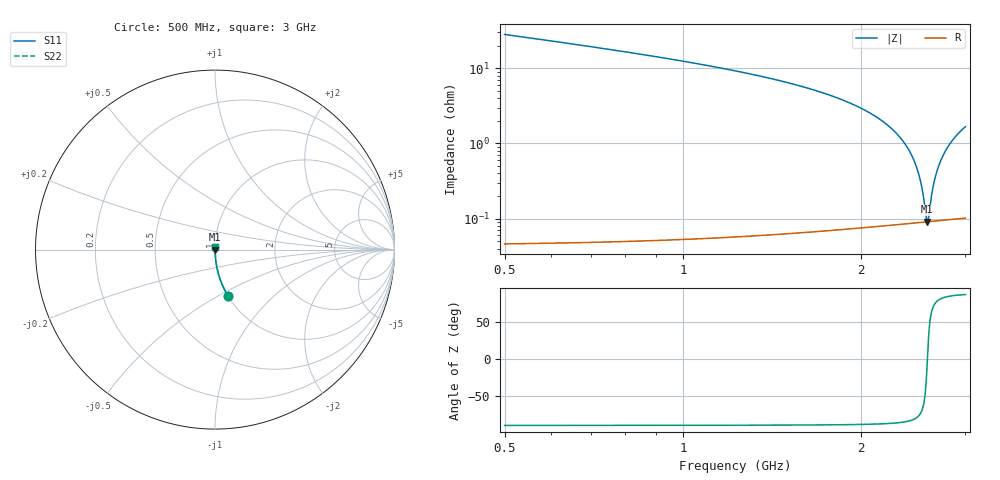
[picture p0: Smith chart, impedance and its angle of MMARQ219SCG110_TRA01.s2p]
! MMARQ219SCG110_TRA01  S-PARAMETER MODEL  ( General Type )
! Model Generated by TAIYO YUDEN Corporation (http://www.ty-top.com)
! Version 1.0
! TAIYO YUDEN Control No. 180601
! Copyright(c) 2018 TAIYO YUDEN CO.,LTD. All Rights Reserved.
! Product Description (link to TY-COMPAS)
! https://ds.yuden.co.jp/TYCOMPAS/or/detail?pn=MMARQ219SCG110JTRA01&u=M
! Products Name : Multilayer Ceramic Capacitors
! Characteristics :
!  Capacitance : 11 pF , Rated Voltage : 250V , TCC : CG / C0G
!  Case Size : 2.0 x 1.25 / 0.079 x 0.049 [mm/inch] , Thickness : 0.85 / 0.033 [mm/inch]
!  (Conditions: Temperature = 25 degC , DC Bias Current/Voltage = 0A / 0V)
! External Node Assignments :
!  1  o---| |---o  2
! GND o---------o GND
! Frequency Range : 500MHz  -  3000MHz  [ 401 STEP ]
# MHz S RI R 50
! Freq[MHz].  S11 Real  S11 Imag  S21 Real  S21 Imag  S12 Real  S12 Imag  S22 Real  S22 Imag
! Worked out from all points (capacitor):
!   401 points, 500 MHz to 3 GHz, reference 50 ohm
!   read as one part in series: C = 10.9 pF near 512.5 MHz
!   lowest |Z| = 90.7 mohm at 2.587 GHz (marker M1)
!   series resonance near 2.588 GHz, so ESL is about 350 pH
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500  0.0736 -0.2604  0.9264 0.2604  0.9264 0.2604  0.0736 -0.2604
918.75  0.0194 -0.1361  0.9806 0.1361  0.9806 0.1361  0.0194 -0.1361
1337.5  0.00693 -0.0793  0.9931 0.0793  0.9931 0.0793  0.00693 -0.0793
1750  0.00272 -0.0451  0.9973 0.0451  0.9973 0.0451  0.00272 -0.0451
1987.5  0.00165 -0.03  0.9984 0.03  0.9984 0.03  0.00165 -0.03
2168.75  0.00119 -0.02  0.9988 0.02  0.9988 0.02  0.00119 -0.02
2337.5  0.000971 -0.0115  0.999 0.0115  0.999 0.0115  0.000971 -0.0115
2400  0.000928 -0.00848  0.9991 0.00848  0.9991 0.00848  0.000928 -0.00848
2450  0.000907 -0.00616  0.9991 0.00616  0.9991 0.00616  0.000907 -0.00616
2487.5  0.000899 -0.00445  0.9991 0.00445  0.9991 0.00445  0.000899 -0.00445
2518.75  0.000897 -0.00305  0.9991 0.00305  0.9991 0.00305  0.000897 -0.00305
2543.75  0.000898 -0.00194  0.9991 0.00194  0.9991 0.00194  0.000898 -0.00194
2575  0.000903 -0.00057  0.9991 0.00057  0.9991 0.00057  0.000903 -0.00057
2587.5  0.000906 -2.67e-05  0.9991 2.67e-05  0.9991 2.67e-05  0.000906 -2.67e-05
2600  0.00091 0.000514  0.9991 -0.000514  0.9991 -0.000514  0.00091 0.000514
2631.25  0.000921 0.00186  0.9991 -0.00186  0.9991 -0.00186  0.000921 0.00186
2656.25  0.000933 0.00292  0.9991 -0.00292  0.9991 -0.00292  0.000933 0.00292
2687.5  0.000951 0.00423  0.999 -0.00423  0.999 -0.00423  0.000951 0.00423
2725  0.000976 0.00579  0.999 -0.00579  0.999 -0.00579  0.000976 0.00579
2775  0.00102 0.00783  0.999 -0.00783  0.999 -0.00783  0.00102 0.00783
2837.5  0.00108 0.0103  0.9989 -0.0103  0.9989 -0.0103  0.00108 0.0103
3000  0.00129 0.0166  0.9987 -0.0166  0.9987 -0.0166  0.00129 0.0166
